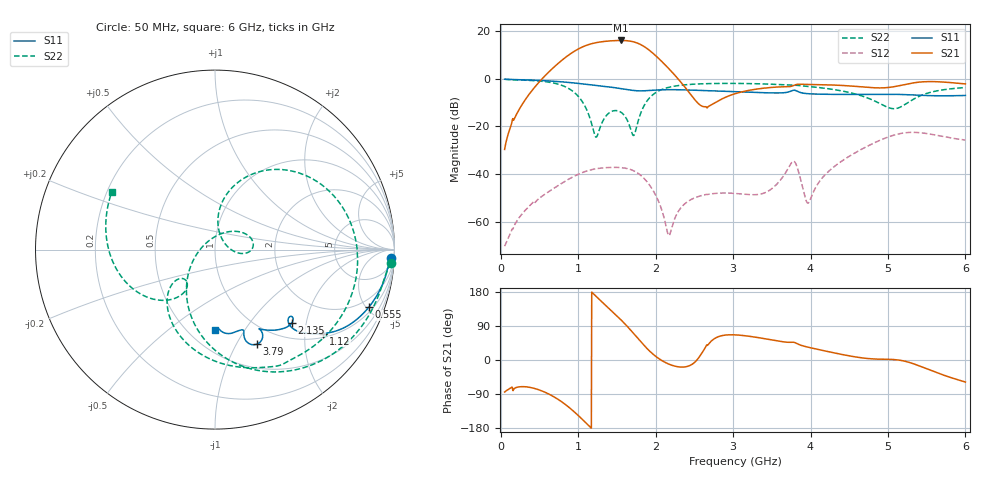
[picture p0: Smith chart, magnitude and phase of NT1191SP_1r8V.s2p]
! Created Wed Apr  6 17:07:04 2022
# hz S ma R 50
! 2 Port Network Data from SP4.SP block
! freq  magS11  angS11  magS21  angS21  magS12  angS12  magS22  angS22
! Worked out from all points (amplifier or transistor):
!   1191 points, 50 MHz to 6 GHz, reference 50 ohm
!   highest |S21| = 16.1 dB at 1.55 GHz (marker M1)
!   |S21| within 3 dB of that: 1.037 GHz to 1.872 GHz (835.3 MHz wide, 57.4 % of centre)
!   unconditionally stable (mu >= 1): start of sweep to end of sweep
!   at 1.04 GHz: K = 3.49, MAG = 18.0 dB, |S12| = -39.5 dB
!   at 3.025 GHz: K = 67.16, MAG = -0.4 dB, |S12| = -48.1 dB
!   at 6 GHz: K = 5.41, MAG = 1.5 dB, |S12| = -25.7 dB
!   lowest NFmin = 0.59 dB at 870 MHz
!   S11 on the Smith chart (normalised r, x): 50 MHz: 15, -37; 555 MHz: 1.32, -5.21; 1.12 GHz: 1.11, -2.48; 2.135 GHz: 1.32, -1.65; 3.79 GHz: 0.77, -1.22; 6 GHz: 0.67, -0.75
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5e7  0.9817 -2.7  0.03295 -84.6  0.0003073 -65.8  0.9812 -4.5
5.55e8  0.9154 -20.5  1.086 -83.6  0.003636 153.6  0.8796 -40.8
7.95e8  0.8626 -28.6  2.495 -111.4  0.006523 128.7  0.7238 -69.1
9.3e8  0.8238 -32.9  3.609 -133.4  0.008715 113.9  0.549 -91.3
1.045e9  0.7866 -36.1  4.588 -155.0  0.01065 99.7  0.3476 -115.6
1.12e9  0.7619 -37.9  5.14 -169.9  0.01176 89.6  0.2062 -136.7
1.22e9  0.7304 -40.0  5.69 170.2  0.01285 76.0  0.06247 148.3
1.325e9  0.6986 -42.0  6.06 149.9  0.01354 61.9  0.1364 48.1
1.435e9  0.664 -43.9  6.287 129.0  0.01383 46.8  0.2078 19.1
1.55e9  0.6237 -45.3  6.386 106.5  0.01369 29.6  0.2 -1.2
1.675e9  0.5799 -45.0  6.171 79.4  0.0125 7.6  0.0908 -0.5
1.805e9  0.5588 -42.4  5.251 48.9  0.009502 -18.7  0.1855 84.6
1.9e9  0.5664 -41.1  4.195 28.0  0.006551 -37.7  0.3623 74.2
2.035e9  0.5845 -41.9  2.717 4.6  0.002751 -63.7  0.5526 53.9
2.135e9  0.5912 -43.6  1.876 -7.6  0.0007993 -103.3  0.6407 41.2
2.465e9  0.5795 -49.5  0.4424 -12.1  0.002966 109.1  0.767 12.3
3.025e9  0.5341 -57.1  0.4863 66.3  0.003928 105.6  0.8012 -19.3
3.79e9  0.5763 -66.1  0.7334 46.5  0.01844 116.6  0.74 -60.4
3.95e9  0.49 -70.8  0.7631 34.7  0.002619 113.7  0.6966 -70.9
4.02e9  0.4819 -70.5  0.7594 31.4  0.003626 174.2  0.6793 -75.4
5.01e9  0.4747 -79.9  0.6591 1.8  0.06067 149.4  0.2477 -139.6
6e9  0.4469 -89.9  0.7814 -58.1  0.05183 75.3  0.6583 151.0
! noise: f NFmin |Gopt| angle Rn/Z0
5e+07  4.2  0.9727  2.812  35.69
7.1e+08  0.5972  0.7412  21.15  0.4117
1.37e+09  0.6446  0.6639  37.06  0.3132
2.03e+09  1  0.5821  52.28  0.3171
2.69e+09  6.903  0.5502  54.44  2.864
3.355e+09  3.324  0.4335  68.89  0.6523
4.015e+09  3.564  0.3814  81.47  0.5811
4.675e+09  5.212  0.3502  81.88  0.952
5.335e+09  4.783  0.2694  102.4  0.634
6e+09  4.789  0.1834  108.3  0.6055
